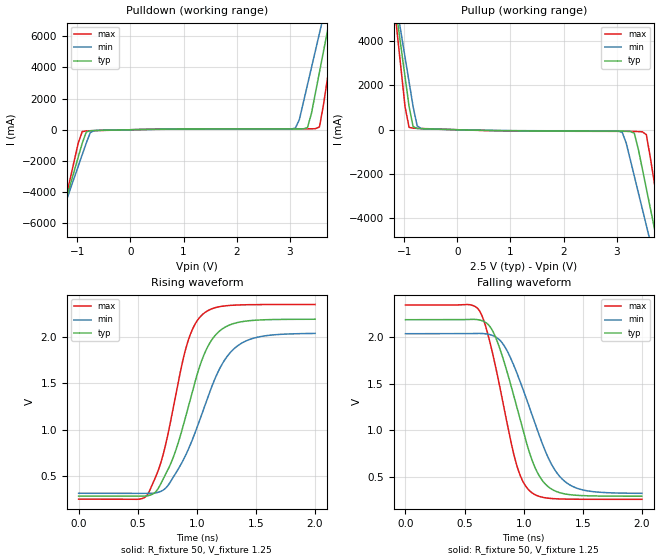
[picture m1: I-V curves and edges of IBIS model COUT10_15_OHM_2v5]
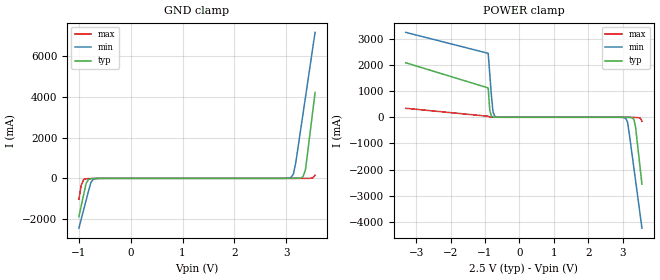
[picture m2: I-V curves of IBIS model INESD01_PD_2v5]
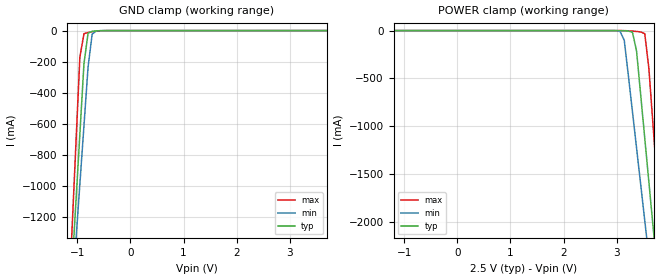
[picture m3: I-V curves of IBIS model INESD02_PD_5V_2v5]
|   This file is an IBIS representation of the   |
|   Integrated Device Technology, Inc.   |
|   ICS87608i   |
|   LOW VOLTAGE/LOW SKEW, 1:8 PCI/PCI-X ZERO DELAY CLOCK GENERATOR   |
[IBIS Ver]   4.1
[File name]   87608i.ibs
[File Rev]   1.0
[Date]   22 Jun 2009 | Last modified
[Source]   Originated at Integrated Device Technology, Inc.
[Disclaimer]
IDT hereby grants the user of this IBIS model a non-exclusive,
nontransferable license to use this IBIS model under the following terms.
Before using this IBIS model, the user should read this license.
If the user does not accept these terms,  the IBIS model should be
returned to IDT within 30 days.
   The user is granted this license only to use the IBIS model and
is not granted rights to sell, load, rent, lease or license the IBIS
model in whole or in part, or in modified form to anyone other than
user. User may modify the IBIS model to suit its specific
applications but rights to derivative works and such modifications
shall belong to IDT.
   This IBIS model is provided on an "AS IS" basis and IDT makes
absolutely no warranty with respect to the information contained
herein. IDT DISCLAIMS AND CUSTOMER WAIVES ALL WARRANTIES, EXPRESS
OR IMPLIED, INCLUDING WARRANTIES OF MERCHANTABILITY OR FITNESS FOR
A PARTICULAR PURPOSE. The entire risk as to quality and performance
is with the Customer. ACCORDINGLY, IN NO EVENT SHALL THE COMPANY BE
LIABLE FOR ANY DAMAGES, WHETHER IN CONTRACT OR TORT,INCLUDING ANY
LOST PROFITS OR OTHER INCIDENTAL, CONSEQUENTIAL, EXEMPLARY, OR
PUNITIVE DAMAGES ARISING OUT OF THE USE OR APPLICATION OF THE IBIS
model provided in this package. Further, IDT reserves the right to
make changes without notice to any product herein to improve
reliability, function, or design. IDT does not convey any license
under patent rights or any other intellectual property rights,
including those of third parties.
   IDT is not obligated to provide maintenance or support
for the licensed IBIS model.
[Copyright]   Copyright 2007 by Integrated Device Technology, Inc.
[Component]   ICS87608YI
[Manufacturer] Integrated Device Technology, Inc.
[Package]
|LQFP32
|lead + wire   typ   min   max
R_pkg   220.4m   212.5m   238m
L_pkg   1.841n   1.708n   1.974n
C_pkg   0.316p   0.2907p   0.33p
[Pin] signal_name  model_name   R_pin   L_pin   C_pin
1   QA0   COUT10_15_OHM   238m   1.974n   0.330p
2   QA1   COUT10_15_OHM   225m   1.841n   0.311p
3   GND   GND   218m   1.7745n   0.301p
4   QA2   COUT10_15_OHM   213m   1.708n   0.291p
5   QA3   COUT10_15_OHM   213m   1.708n   0.291p
6   VDDOA   POWER   218m   1.7745n   0.301p
7   MR   INESD01_PD   225m   1.841n   0.311p
8   DIV_SELA0   INESD01_PD   238m   1.974n   0.330p
9   DIV_SELA1   INESD01_PD   238m   1.974n   0.330p
10  DIV_SELB0   INESD01_PD   225m   1.841n   0.311p
11  DIV_SELB1   INESD01_PD   218m   1.7745n   0.301p
12  FBDIV_SEL0  INESD01_PD   213m   1.708n   0.291p
13  FBDIV_SEL1  INESD01_PD   213m   1.708n   0.291p
14  VDD   POWER   218m   1.7745n   0.301p
15  FB_IN   INESD02_PD_5V   225m   1.841n   0.311p
16  GND   GND   238m   1.974n   0.330p
17  FB_OUT   COUT10_15_OHM   238m   1.974n   0.330p
18  REF_OUT   COUT10_15_OHM   225m   1.841n   0.311p
19  VDDOB   POWER   218m   1.7745n   0.301p
20  QB3   COUT10_15_OHM   213m   1.708n   0.291p
21  QB2   COUT10_15_OHM   213m   1.708n   0.291p
22  GND   GND   218m   1.7745n   0.301p
23  QB1   COUT10_15_OHM   225m   1.841n   0.311p
24  QB0   COUT10_15_OHM   238m   1.974n   0.330p
25  VDDOB   POWER   238m   1.974n   0.330p
26  PLL_SEL   INESD01_PU   225m   1.841n   0.311p
27  VDDA   POWER   218m   1.7745n   0.301p
28  XTAL_SEL   INESD01_PU   213m   1.708n   0.291p
29  XTAL1   NC   213m   1.708n   0.291p
30  XTAL2   NC   218m   1.7745n   0.301p
31  REF_IN   INESD02_PD_5V   225m   1.841n   0.311p
32  VDDOA   POWER   238m   1.974n   0.330p
[Model Selector] COUT10_15_OHM
COUT10_15_OHM_2v5  Buffer selection for 2v5
COUT10_15_OHM_3v3  Buffer selection for 3v3
[Model Selector] INESD01_PD
INESD01_PD_2v5  Buffer selection for 2v5
INESD01_PD_3v3  Buffer selection for 3v3
[Model Selector] INESD02_PD_5V
INESD02_PD_5V_2v5  Buffer selection for 2v5
INESD02_PD_5V_3v3  Buffer selection for 3v3
[Model Selector] INESD01_PU
INESD01_PU_2v5  Buffer selection for 2v5
INESD01_PU_3v3  Buffer selection for 3v3
| Models and submodels in the file (8): COUT10_15_OHM_2v5 (Output), INESD01_PD_2v5 (Input), INESD02_PD_5V_2v5 (Input), INESD01_PU_2v5 (Input), COUT10_15_OHM_3v3 (Output), INESD01_PD_3v3 (Input), INESD02_PD_5V_3v3 (Input), INESD01_PU_3v3 (Input)
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[Model] COUT10_15_OHM_2v5
Model_type   Output
Polarity   Non-Inverting
|   typ   min   max
C_comp   2pF   1.5pF   2.5pF
Vmeas = 1.25V
Rref = 50
Cref = 0
Vref = 1.25V
|   typ   min   max
[Voltage range]   2.5V   2.375V   2.625V
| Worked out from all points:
|   slope of the pulldown table from 0 to 0.375 V, typ, clamps not added: 15.7 ohm
|   slope of the pullup table from 0 to 0.375 V, typ, clamps not added: 16.9 ohm
|   rising waveform, R_fixture 50, V_fixture 1.25: 20-80 % time 271ps typ, 328ps min, 218ps max; typ from 0.289 V to 2.19 V
|   falling waveform, R_fixture 50, V_fixture 1.25: 20-80 % time 257ps typ, 305ps min, 212ps max; typ from 2.19 V to 0.289 V
[Pulldown]
|Voltage   I (typ)   I (min)   I (max)
-2.5V     -19.68A    -17.28A    -23.73A
-1.439V   -7.139A    -6.83A     -7.73A
-1.364V   -6.243A    -6.083A    -6.586A
-909.1mV  -868mA     -1.604A    -120mA
-833.3mV  -148.1mA   -858.1mA   -77.34mA
-681.8mV  -50.66mA   -56.35mA   -57.61mA
3.106V    52.05mA    102mA      60.73mA
3.333V    133.3mA    2.872A     61.18mA
3.561V    3.704A     6.201A     183.5mA
3.712V    6.369A     8.421A     3.314A
3.864V    9.036A     10.64A     6.72A
5V        29.06A     27.33A     32.31A
[Pullup]
|Voltage   I (typ)   I (min)   I (max)
-2.5V     29.11A     25.53A     35.17A
-1.136V   5.055A     5.495A     4.444A
-909.1mV  1.05A      2.158A     108.2mA
-833.3mV  137.8mA    1.047A     70.3mA
-681.8mV  48.38mA    53.62mA    56.56mA
3.106V    -62.59mA   -118.3mA   -71.54mA
3.333V    -157.8mA   -2.094A    -77.62mA
3.485V    -1.769A    -3.583A    -93.66mA
3.561V    -2.662A    -4.328A    -221.8mA
3.712V    -4.451A    -5.818A    -2.414A
3.864V    -6.24A     -7.309A    -4.698A
5V        -19.66A    -18.5A     -21.84A
[Ramp]
|   typ   min   max
dV/dt_r   1.522/0.426n   1.376/0.508n   1.676/0.344n
dV/dt_f   1.524/0.384n   1.378/0.458n   1.679/0.314n
R_load =   50.0000
[Rising Waveform]
R_fixture = 50
V_fixture = 1.25   |Vcc_typ
V_fixture_min = 1.1875 |Vcc_min
V_fixture_max = 1.3125 |Vcc_max
C_fixture = 0.0p
| Time   typ   min   max
0s        288.7mV    318.6mV    255.3mV
584.6ps   292.1mV    317.4mV    308.2mV
696.7ps   424.5mV    339.9mV    652.6mV
790.8ps   672.5mV    470.8mV    1.172V
922.9ps   1.225V     775.3mV    1.945V
1.057ns   1.797V     1.223V     2.251V
1.205ns   2.076V     1.688V     2.328V
1.357ns   2.158V     1.915V     2.344V
1.574ns   2.184V     2.011V     2.348V
2ns       2.19V      2.038V     2.349V
[Falling Waveform]
R_fixture = 50
V_fixture = 1.25   |Vcc_typ
V_fixture_min = 1.1875 |Vcc_min
V_fixture_max = 1.3125 |Vcc_max
C_fixture = 0.0p
| Time   typ   min   max
0s        2.19V      2.04V      2.349V
532.5ps   2.193V     2.04V      2.353V
624.6ps   2.188V     2.043V     2.289V
688.7ps   2.151V     2.037V     2.071V
778.8ps   1.948V     1.991V     1.585V
936.9ps   1.272V     1.633V     640.5mV
1.061ns   712mV      1.2V       334.7mV
1.183ns   419.5mV    773.5mV    271.8mV
1.363ns   310.3mV    432.8mV    257.5mV
2ns       288.9mV    319.9mV    255.3mV
[Model] INESD01_PD_2v5
Model_type   Input
Polarity   Non-Inverting
Vinl = 0.8V
Vinh = 2.0V
|   typ   min   max
C_comp   2pF   1.5pF   2.5pF
|   typ   min   max
[Voltage range]  2.5V   2.375V   2.625V
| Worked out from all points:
|   GND clamp passes 1 mA (typ) near -0.55 V on its own axis
|   POWER clamp passes 1 mA (typ) near -0.68 V on its own axis
[GND_clamp]
|Voltage I(typ)   I(min)   I(max)
-1V       -1.886A    -2.451A    -1.028A
-953.5mV  -1.338A    -1.994A    -328mA
-907mV    -789.6mA   -1.537A    -53.04mA
-860.5mV  -251.4mA   -1.081A    -21.51mA
-767.5mV  -17.28mA   -198.8mA   -10.01mA
-674.5mV  -5.28mA    -15.38mA   -3.684mA
3.092V    224.5uA    49.06mA    51.52uA
3.139V    500.8uA    208.3mA    52.98uA
3.185V    1.252mA    774.6mA    56.66uA
3.325V    81.55mA    3.177A     200uA
3.371V    416.9mA    3.978A     464.6uA
3.557V    4.225A     7.185A     159.2mA
[POWER_clamp]
|Voltage   I(typ)   I(min)   I(max)
-3.3V     2.083A     3.246A     343.1mA
-907mV    1.122A     2.445A     37.78mA
-860.5mV  267.5mA    1.644A     5.973mA
-814mV    47.03mA    844mA      1.727mA
-767.5mV  9.66mA     215.3mA    677uA
-674.5mV  960.6uA    12.66mA    131.4uA
3.092V    -1.849mA   -49.09mA   -51.51uA
3.139V    -3.491mA   -186mA     -159.7uA
3.325V    -84.03mA   -1.955A    -5.102mA
3.371V    -365.4mA   -2.411A    -8.31mA
3.51V     -2.01A     -3.782A    -35.44mA
3.557V    -2.558A    -4.239A    -152.3mA
[Model] INESD02_PD_5V_2v5
Model_type   Input
Polarity   Non-Inverting
Vinl = .87V
Vinh = 1.62V
|   typ   min   max
C_comp   2pF   1.5pF   2.5pF
|   typ   min   max
[Voltage range]   2.5V   2.375V   2.625V
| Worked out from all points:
|   GND clamp passes 1 mA (typ) near -0.59 V on its own axis
[GND_clamp]
|Voltage   I(typ)   I(min)   I(max)
-2.191V   -7.973A    -7.07A     -9.504A
-1.108V   -1.581A    -1.751A    -1.338A
-1.031V   -1.125A    -1.371A    -755.2mA
-953.6mV  -669.5mA   -992.5mA   -172.1mA
-876.3mV  -213.9mA   -613.7mA   -19.96mA
-799mV    -17.31mA   -235.3mA   -12.11mA
-721.6mV  -4.455mA   -23.01mA   -7.724mA
-644.3mV  -1.863mA   -2.522mA   -4.06mA
5V        97.41uA    121.8uA    75.48uA
[POWER_clamp]
|Voltage   I(typ)   I(min)   I(max)
-2.5V     97.41uA    118.8uA    77.37uA
2.835V    -9.233uA   -44.7uA    -3.208uA
3.067V    -617.5uA   -9.489mA   -116.3uA
3.144V    -1.863mA   -101.8mA   -642.8uA
3.299V    -17.31mA   -847.2mA   -5.362mA
3.376V    -213.9mA   -1.226A    -9.326mA
3.531V    -1.125A    -1.985A    -32.65mA
3.608V    -1.581A    -2.364A    -395.6mA
3.686V    -2.038A    -2.744A    -978.8mA
3.763V    -2.494A    -3.124A    -1.562A
3.84V     -2.95A     -3.503A    -2.145A
4.845V    -8.886A    -8.445A    -9.728A
